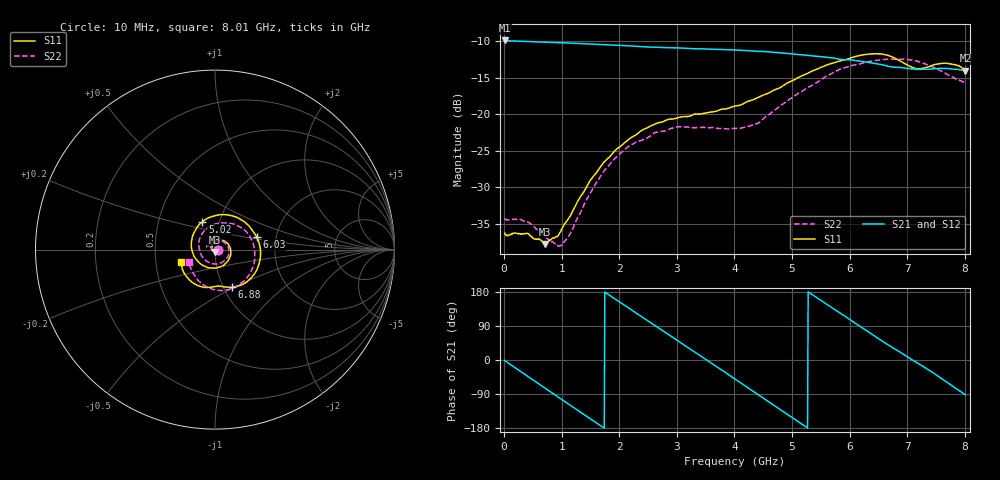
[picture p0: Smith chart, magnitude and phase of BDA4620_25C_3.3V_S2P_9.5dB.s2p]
!Agilent Technologies,E5071B,MY42404982,A.09.10
!Date: Wed May 06 08:50:26 2026
!Data & Calibration Information:
!Freq	S11:SOLT2(ON)	S21:SOLT2(ON)	S12:SOLT2(ON)	S22:SOLT2(ON)
# Hz S RI R 50
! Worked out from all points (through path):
!   801 points, 10 MHz to 8.01 GHz, reference 50 ohm
!   highest |S21| = -9.94 dB at 10 MHz (marker M1); lowest = -14.1 dB at 8.01 GHz (marker M2)
!   group delay of S21, straight-line fit = 281 ps
!   lowest |S11| = -37.7 dB at 710 MHz (marker M3), VSWR 1.03, Z = 49.9 - j1.3 ohm
!   |S11| at or under -10 dB: start of sweep to end of sweep
!   |S22| runs from -38.0 to -12.5 dB; largest |S21 - S12| = 0.0013
!   S11 on the Smith chart (normalised r, x): 10 MHz: 1.03, -0.00; 5.02 GHz: 0.83, +0.27; 6.03 GHz: 1.58, +0.24; 6.88 GHz: 1.10, -0.49; 8.01 GHz: 0.68, -0.10
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1e7  0.0154 -0.00106  0.3182 -0.00694  0.3187 -0.00696  0.0195 -0.00116
3.3e8  0.0124 -0.00883  0.2582 -0.1786  0.2586 -0.179  0.0165 -0.00901
7.1e8  -0.00117 -0.013  0.0853 -0.2985  0.0852 -0.2991  0.00307 -0.0144
9.9e8  -0.015 -0.00563  -0.0687 -0.2993  -0.069 -0.2999  -0.0101 -0.0078
1.35e9  -0.0214 0.0183  -0.2319 -0.195  -0.2321 -0.1951  -0.0176 0.0136
1.65e9  -0.00856 0.0415  -0.2948 -0.0488  -0.2953 -0.049  -0.00887 0.0352
1.94e9  0.0182 0.054  -0.2772 0.1017  -0.2777 0.1021  0.0136 0.0487
2.32e9  0.0606 0.042  -0.1497 0.2486  -0.1501 0.2488  0.0503 0.0415
2.68e9  0.0874 0.000972  0.0254 0.2846  0.0258 0.2849  0.0744 0.0124
2.99e9  0.0812 -0.0471  0.1682 0.2281  0.1688 0.2281  0.0779 -0.0245
3.39e9  0.034 -0.094  0.2718 0.0632  0.2725 0.0629  0.0447 -0.0675
4.01e9  -0.0823 -0.0782  0.1751 -0.2104  0.1753 -0.2109  -0.0505 -0.062
4.5e9  -0.1325 0.026  -0.0485 -0.2633  -0.0488 -0.2639  -0.0905 0.021
5.02e9  -0.0698 0.155  -0.2309 -0.1138  -0.2315 -0.1138  -0.032 0.1274
5.35e9  0.0307 0.1947  -0.2476 0.0317  -0.2479 0.0318  0.0521 0.1486
6.03e9  0.2325 0.0702  -0.057 0.2273  -0.057 0.2277  0.2106 0.0396
6.36e9  0.2484 -0.0679  0.0748 0.2115  0.075 0.2117  0.2202 -0.064
6.68e9  0.1695 -0.1851  0.1648 0.1327  0.1656 0.1331  0.1757 -0.1599
6.88e9  0.0955 -0.2099  0.1955 0.0719  0.196 0.0721  0.1249 -0.2015
7.18e9  0.0191 -0.2032  0.2 -0.0287  0.2006 -0.029  0.0244 -0.2278
7.56e9  -0.0848 -0.2038  0.1449 -0.1454  0.1453 -0.1457  -0.0841 -0.1808
8.01e9  -0.1876 -0.0711  -0.00635 -0.1982  -0.00622 -0.1986  -0.1459 -0.0712
